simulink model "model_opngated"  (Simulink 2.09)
settings: Solver=ode1  StartTime=0.0  StopTime=1  FixedStep=0.001  MaxStep=0.001  RelTol=1e-5  AbsTol=1e-6
undefined symbols (not defined in the file or in its folder): movedetect

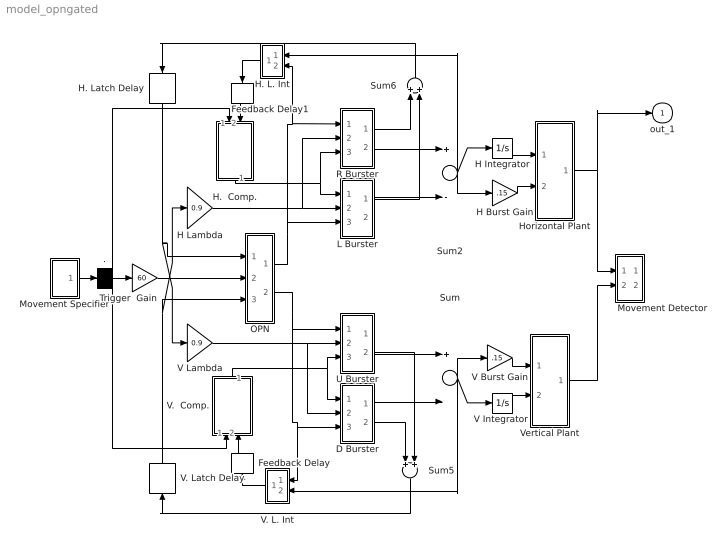
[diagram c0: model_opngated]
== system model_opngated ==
  . : Demux  Outputs=3
  D Burster : Subsystem
  Feedback Delay : TransportDelay  Orientation=up  DelayTime=.005  InitialInput=00  BufferSize=1024
  Feedback Delay1 : TransportDelay  Orientation=down  DelayTime=.005  InitialInput=00  BufferSize=1024
  H Burst Gain : Gain  Gain=.15
  H Integrator : Integrator  ExternalReset=none  InitialConditionSource=internal  InitialCondition=0  LimitOutput=off  UpperSaturationLimit=inf  LowerSaturationLimit=-inf  ShowSaturationPort=off  ShowStatePort=off  AbsoluteTolerance=auto
  H Lambda : Gain  Gain=0.9
  H.  Comp. : Subsystem  Orientation=down
  H. L. Int : Subsystem  Orientation=left
  H. Latch Delay : TransportDelay  Orientation=down  DelayTime=0  InitialInput=00  BufferSize=1024
  Horizontal Plant : Subsystem
  L Burster : Subsystem
  Movement Detector : Subsystem
  Movement Specifier : Subsystem
  OPN : Subsystem
  R Burster : Subsystem
  Sum : Sum  Inputs=+-
  Sum2 : Sum  Inputs=+-
  Sum5 : Sum  Orientation=down  Inputs=++
  Sum6 : Sum  Orientation=up  Inputs=++
  Trigger  Gain : Gain  Gain=60
  U Burster : Subsystem
  V Burst Gain : Gain  Gain=.15
  "V Integrator " : Integrator  ExternalReset=none  InitialConditionSource=internal  InitialCondition=0  LimitOutput=off  UpperSaturationLimit=inf  LowerSaturationLimit=-inf  ShowSaturationPort=off  ShowStatePort=off  AbsoluteTolerance=auto
  V Lambda : Gain  Gain=0.9
  V.  Comp. : Subsystem  Orientation=up
  V. L. Int : Subsystem  Orientation=left
  V. Latch Delay : TransportDelay  Orientation=up  DelayTime=0  InitialInput=00  BufferSize=1024
  Vertical Plant : Subsystem
  out_1 : Outport  Port=1  InitialOutput=0
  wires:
  OPN/1(out_1) -> H. L. Int/2(OPN Input), R Burster/1(in_3), L Burster/3(in_3)
  Horizontal Plant/1(out_1) -> out_1/1, Movement Detector/1(Horizontal Position)
  ./3 -> V.  Comp./1(in_4)
  Movement Specifier/1(out_1) -> ./1
  ./1 -> H.  Comp./1(in_1)
  ./2 -> Trigger  Gain/1
  Vertical Plant/1(out_1) -> Movement Detector/2(Veritcal Position)
  H Integrator/1 -> Horizontal Plant/1(in_1)
  OPN/2(out_4) -> V. L. Int/1(OPN Input), D Burster/3(in_3), U Burster/1(in_3)
  H. Latch Delay/1 -> V Lambda/1, OPN/1(in_1)
  V. Latch Delay/1 -> H Lambda/1, OPN/3(in_3)
  Trigger  Gain/1 -> OPN/2(in_2)
  R Burster/1(out_2) -> Sum6/1
  Sum5/1 -> V. Latch Delay/1
  Sum6/1 -> H. Latch Delay/1
  L Burster/1(out_1) -> Sum6/2
  V.  Comp./1(out_1) -> D Burster/1(in_1), U Burster/3(in_1)
  V Lambda/1 -> D Burster/2(in_2), U Burster/2(in_2)
  D Burster/1(out_2) -> Sum/2
  D Burster/2(out_3) -> Sum5/1
  U Burster/1(out_3) -> Sum/1
  U Burster/2(out_4) -> Sum5/2
  H Lambda/1 -> R Burster/2(in_2), L Burster/2(in_2)
  R Burster/2(out_3) -> Sum2/1
  L Burster/2(out_2) -> Sum2/2
  H.  Comp./1(out_1) -> R Burster/3(in_1), L Burster/1(in_1)
  Sum/1 -> V. L. Int/2(BURST Input), "V Integrator "/1, V Burst Gain/1
  "V Integrator "/1 -> Vertical Plant/2(in_2)
  V Burst Gain/1 -> Vertical Plant/1(in_1)
  Sum2/1 -> H. L. Int/1(BURST Input), H Burst Gain/1, H Integrator/1
  H Burst Gain/1 -> Horizontal Plant/2(in_2)
  V. L. Int/1(out_1) -> Feedback Delay/1
  Feedback Delay/1 -> V.  Comp./2(in_5)
  H. L. Int/1(out_1) -> Feedback Delay1/1
  Feedback Delay1/1 -> H.  Comp./2(in_2)

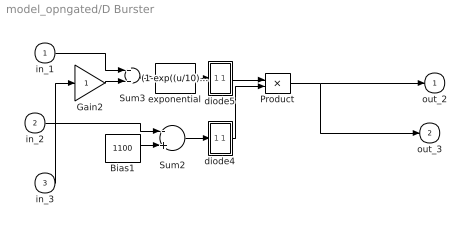
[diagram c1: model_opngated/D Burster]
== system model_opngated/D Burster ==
  in_1 : Inport  Port=1  PortWidth=-1  SampleTime=-1
  in_2 : Inport  Port=2  PortWidth=-1  SampleTime=-1
  in_3 : Inport  Port=3  PortWidth=-1  SampleTime=-1
  Bias1 : Constant  Value=1100
  Gain2 : Gain  Gain=1
  Product : Product  Inputs=2
  Sum2 : Sum  Inputs=-+
  Sum3 : Sum  Inputs=++
  diode4 : Subsystem
  diode5 : Subsystem
  exponential : Fcn  Expr=(1-exp((u/10)))
  out_2 : Outport  Port=1  InitialOutput=0
  out_3 : Outport  Port=2  InitialOutput=0
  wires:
  Product/1 -> out_3/1, out_2/1
  in_3/1 -> Gain2/1
  diode5/1(out_1) -> Product/1
  exponential/1 -> diode5/1(in_1)
  diode4/1(out_1) -> Product/2
  Sum2/1 -> diode4/1(in_1)
  in_2/1 -> Sum2/1
  Bias1/1 -> Sum2/2
  Sum3/1 -> exponential/1
  in_1/1 -> Sum3/1
  Gain2/1 -> Sum3/2

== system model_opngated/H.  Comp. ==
  in_1 : Inport  Port=1  PortWidth=-1  SampleTime=-1
  in_2 : Inport  Port=2  PortWidth=-1  SampleTime=-1
  Sum : Sum  Inputs=+-
  out_1 : Outport  Port=1  InitialOutput=0
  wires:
  in_2/1 -> Sum/2
  in_1/1 -> Sum/1
  Sum/1 -> out_1/1

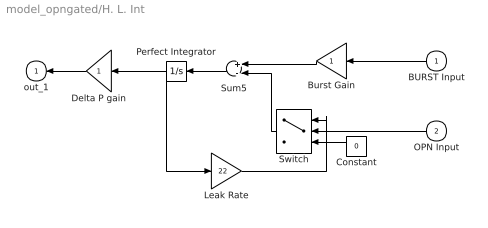
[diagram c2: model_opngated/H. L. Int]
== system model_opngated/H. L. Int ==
  BURST Input : Inport  Orientation=left  Port=1  PortWidth=-1  SampleTime=-1
  OPN Input : Inport  Orientation=left  Port=2  PortWidth=-1  SampleTime=-1
  Burst Gain : Gain  Orientation=left  Gain=1
  Constant : Constant  Orientation=left  Value=0
  Delta P gain : Gain  Orientation=left  Gain=1
  Leak Rate : Gain  Gain=22
  Perfect Integrator : Integrator  Orientation=left  ExternalReset=none  InitialConditionSource=internal  InitialCondition=0  LimitOutput=off  UpperSaturationLimit=inf  LowerSaturationLimit=-inf  ShowSaturationPort=off  ShowStatePort=off  AbsoluteTolerance=auto
  Sum5 : Sum  Orientation=left  Inputs=+-
  Switch : Switch  Orientation=left  Threshold=50
  out_1 : Outport  Orientation=left  Port=1  InitialOutput=0
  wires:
  Switch/1 -> Sum5/2
  Constant/1 -> Switch/3
  Leak Rate/1 -> Switch/1
  Perfect Integrator/1 -> Leak Rate/1, Delta P gain/1
  OPN Input/1 -> Switch/2
  BURST Input/1 -> Burst Gain/1
  Burst Gain/1 -> Sum5/1
  Delta P gain/1 -> out_1/1
  Sum5/1 -> Perfect Integrator/1

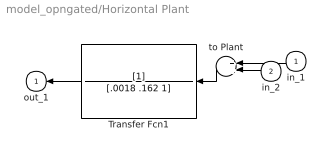
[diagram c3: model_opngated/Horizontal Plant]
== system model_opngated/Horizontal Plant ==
  in_1 : Inport  Orientation=left  Port=1  PortWidth=-1  SampleTime=-1
  in_2 : Inport  Orientation=left  Port=2  PortWidth=-1  SampleTime=-1
  Transfer Fcn1 : TransferFcn  Orientation=left  Numerator=[1]  Denominator=[.0018 .162 1]
  to Plant : Sum  Orientation=left  Inputs=++
  out_1 : Outport  Orientation=left  Port=1  InitialOutput=0
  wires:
  Transfer Fcn1/1 -> out_1/1
  in_2/1 -> to Plant/2
  in_1/1 -> to Plant/1
  to Plant/1 -> Transfer Fcn1/1

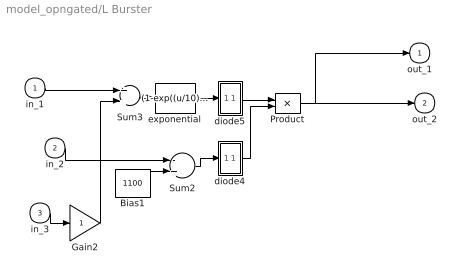
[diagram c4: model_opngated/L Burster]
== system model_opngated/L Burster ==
  in_1 : Inport  Port=1  PortWidth=-1  SampleTime=-1
  in_2 : Inport  Port=2  PortWidth=-1  SampleTime=-1
  in_3 : Inport  Port=3  PortWidth=-1  SampleTime=-1
  Bias1 : Constant  Value=1100
  Gain2 : Gain  Gain=1
  Product : Product  Inputs=2
  Sum2 : Sum  Inputs=-+
  Sum3 : Sum  Inputs=++
  diode4 : Subsystem
  diode5 : Subsystem
  exponential : Fcn  Expr=(1-exp((u/10)))
  out_1 : Outport  Port=1  InitialOutput=0
  out_2 : Outport  Port=2  InitialOutput=0
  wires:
  Product/1 -> out_1/1, out_2/1
  Bias1/1 -> Sum2/2
  in_2/1 -> Sum2/1
  Sum2/1 -> diode4/1(in_1)
  diode4/1(out_1) -> Product/2
  exponential/1 -> diode5/1(in_1)
  diode5/1(out_1) -> Product/1
  Sum3/1 -> exponential/1
  in_3/1 -> Gain2/1
  Gain2/1 -> Sum3/2
  in_1/1 -> Sum3/1

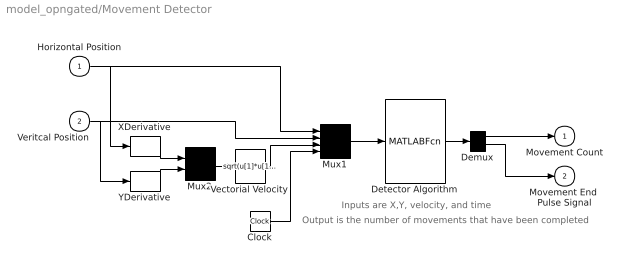
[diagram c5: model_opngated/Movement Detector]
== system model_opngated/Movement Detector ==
  note: Inputs are X,Y, velocity, and time
  note: Output is the number of movements that have been completed
  Horizontal Position : Inport  Port=1  PortWidth=-1  SampleTime=-1
  Veritcal Position : Inport  Port=2  PortWidth=-1  SampleTime=-1
  Clock : Clock
  Demux : Demux  Outputs=2
  Detector Algorithm : MATLABFcn  MATLABFcn=movedetect(u(1),u(2),u(3),u(4))  OutputWidth=2
  Mux1 : Mux  Inputs=4
  Mux2 : Mux  Inputs=2
  Vectorial Velocity : Fcn  Expr=sqrt(u[1]*u[1]+u[2]*u[2])
  XDerivative : Derivative
  YDerivative : Derivative
  Movement Count : Outport  Port=1  InitialOutput=0
  Movement End  Pulse Signal : Outport  Port=2  InitialOutput=0
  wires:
  Demux/2 -> Movement End  Pulse Signal/1
  Demux/1 -> Movement Count/1
  Detector Algorithm/1 -> Demux/1
  Horizontal Position/1 -> XDerivative/1, Mux1/1
  Veritcal Position/1 -> YDerivative/1, Mux1/2
  Vectorial Velocity/1 -> Mux1/3
  Clock/1 -> Mux1/4
  Mux2/1 -> Vectorial Velocity/1
  XDerivative/1 -> Mux2/1
  YDerivative/1 -> Mux2/2
  Mux1/1 -> Detector Algorithm/1

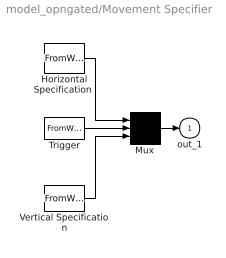
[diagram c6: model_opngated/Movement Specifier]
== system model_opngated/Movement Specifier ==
  "Horizontal Specification " : FromWorkspace  VariableName=hspec
  Mux : Mux  Inputs=3
  Trigger : FromWorkspace  VariableName=trigspec
  Vertical Specification : FromWorkspace  VariableName=vspec
  out_1 : Outport  Port=1  InitialOutput=0
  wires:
  Mux/1 -> out_1/1
  Trigger/1 -> Mux/2
  "Horizontal Specification "/1 -> Mux/1
  Vertical Specification/1 -> Mux/3

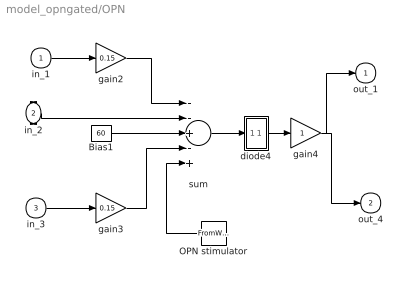
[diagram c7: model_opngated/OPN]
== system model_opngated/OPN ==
  in_1 : Inport  Port=1  PortWidth=-1  SampleTime=-1
  in_2 : Inport  Port=2  PortWidth=-1  SampleTime=-1
  in_3 : Inport  Port=3  PortWidth=-1  SampleTime=-1
  Bias1 : Constant  Value=60
  OPN stimulator : FromWorkspace  Orientation=left  VariableName=stimulate
  diode4 : Subsystem
  gain2 : Gain  Gain=0.15
  gain3 : Gain  Gain=0.15
  gain4 : Gain  Gain=1
  sum : Sum  Inputs=--+-+
  out_1 : Outport  Port=1  InitialOutput=0
  out_4 : Outport  Port=2  InitialOutput=0
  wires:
  OPN stimulator/1 -> sum/5
  gain4/1 -> out_4/1, out_1/1
  diode4/1(out_1) -> gain4/1
  gain3/1 -> sum/4
  in_3/1 -> gain3/1
  gain2/1 -> sum/1
  in_1/1 -> gain2/1
  Bias1/1 -> sum/3
  in_2/1 -> sum/2
  sum/1 -> diode4/1(in_1)

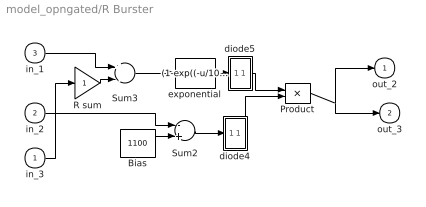
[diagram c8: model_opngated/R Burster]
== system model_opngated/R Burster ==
  in_3 : Inport  Port=1  PortWidth=-1  SampleTime=-1
  in_2 : Inport  Port=2  PortWidth=-1  SampleTime=-1
  in_1 : Inport  Port=3  PortWidth=-1  SampleTime=-1
  Bias : Constant  Value=1100
  Product : Product  Inputs=2
  R sum : Gain  Gain=1
  Sum2 : Sum  Inputs=-+
  Sum3 : Sum  Inputs=+-
  diode4 : Subsystem
  diode5 : Subsystem
  exponential : Fcn  Expr=(1-exp((-u/10)))
  out_2 : Outport  Port=1  InitialOutput=0
  out_3 : Outport  Port=2  InitialOutput=0
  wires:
  in_3/1 -> R sum/1
  Product/1 -> out_3/1, out_2/1
  Bias/1 -> Sum2/2
  in_2/1 -> Sum2/1
  Sum2/1 -> diode4/1(in_1)
  diode4/1(out_1) -> Product/2
  exponential/1 -> diode5/1(in_1)
  diode5/1(out_1) -> Product/1
  R sum/1 -> Sum3/2
  in_1/1 -> Sum3/1
  Sum3/1 -> exponential/1

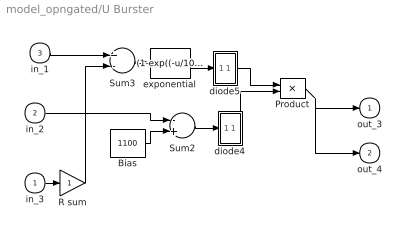
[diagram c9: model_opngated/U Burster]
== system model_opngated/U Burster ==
  in_3 : Inport  Port=1  PortWidth=-1  SampleTime=-1
  in_2 : Inport  Port=2  PortWidth=-1  SampleTime=-1
  in_1 : Inport  Port=3  PortWidth=-1  SampleTime=-1
  Bias : Constant  Value=1100
  Product : Product  Inputs=2
  R sum : Gain  Gain=1
  Sum2 : Sum  Inputs=-+
  Sum3 : Sum  Inputs=+-
  diode4 : Subsystem
  diode5 : Subsystem
  exponential : Fcn  Expr=(1-exp((-u/10)))
  out_3 : Outport  Port=1  InitialOutput=0
  out_4 : Outport  Port=2  InitialOutput=0
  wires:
  Product/1 -> out_3/1, out_4/1
  in_3/1 -> R sum/1
  Bias/1 -> Sum2/2
  in_2/1 -> Sum2/1
  Sum2/1 -> diode4/1(in_1)
  diode4/1(out_1) -> Product/2
  exponential/1 -> diode5/1(in_1)
  diode5/1(out_1) -> Product/1
  in_1/1 -> Sum3/1
  R sum/1 -> Sum3/2
  Sum3/1 -> exponential/1

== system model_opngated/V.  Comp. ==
  in_4 : Inport  Port=1  PortWidth=-1  SampleTime=-1
  in_5 : Inport  Port=2  PortWidth=-1  SampleTime=-1
  Sum : Sum  Inputs=-+
  out_1 : Outport  Port=1  InitialOutput=0
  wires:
  in_4/1 -> Sum/2
  in_5/1 -> Sum/1
  Sum/1 -> out_1/1

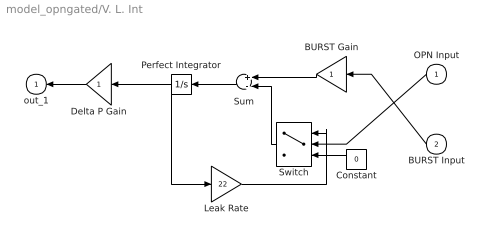
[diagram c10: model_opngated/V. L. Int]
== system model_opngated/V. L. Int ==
  OPN Input : Inport  Orientation=left  Port=1  PortWidth=-1  SampleTime=-1
  BURST Input : Inport  Orientation=left  Port=2  PortWidth=-1  SampleTime=-1
  BURST Gain : Gain  Orientation=left  Gain=1
  Constant : Constant  Orientation=left  Value=0
  Delta P Gain : Gain  Orientation=left  Gain=1
  Leak Rate : Gain  Gain=22
  Perfect Integrator : Integrator  Orientation=left  ExternalReset=none  InitialConditionSource=internal  InitialCondition=0  LimitOutput=off  UpperSaturationLimit=inf  LowerSaturationLimit=-inf  ShowSaturationPort=off  ShowStatePort=off  AbsoluteTolerance=auto
  Sum : Sum  Orientation=left  Inputs=+-
  Switch : Switch  Orientation=left  Threshold=50
  out_1 : Outport  Orientation=left  Port=1  InitialOutput=0
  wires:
  BURST Input/1 -> BURST Gain/1
  OPN Input/1 -> Switch/2
  Sum/1 -> Perfect Integrator/1
  Perfect Integrator/1 -> Delta P Gain/1, Leak Rate/1
  Delta P Gain/1 -> out_1/1
  BURST Gain/1 -> Sum/1
  Leak Rate/1 -> Switch/1
  Constant/1 -> Switch/3
  Switch/1 -> Sum/2

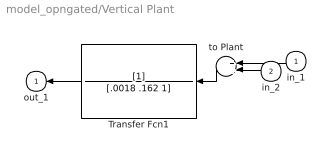
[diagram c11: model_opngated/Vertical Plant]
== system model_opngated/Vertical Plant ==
  in_1 : Inport  Orientation=left  Port=1  PortWidth=-1  SampleTime=-1
  in_2 : Inport  Orientation=left  Port=2  PortWidth=-1  SampleTime=-1
  Transfer Fcn1 : TransferFcn  Orientation=left  Numerator=[1]  Denominator=[.0018 .162 1]
  to Plant : Sum  Orientation=left  Inputs=++
  out_1 : Outport  Orientation=left  Port=1  InitialOutput=0
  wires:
  Transfer Fcn1/1 -> out_1/1
  in_2/1 -> to Plant/2
  in_1/1 -> to Plant/1
  to Plant/1 -> Transfer Fcn1/1

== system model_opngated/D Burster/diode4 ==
  in_1 : Inport  Port=1  PortWidth=-1  SampleTime=-1
  Switch : Switch  Threshold=0
  diode1 : Constant  Value=0
  out_1 : Outport  Port=1  InitialOutput=0
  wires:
  diode1/1 -> Switch/3
  Switch/1 -> out_1/1
  in_1/1 -> Switch/1, Switch/2

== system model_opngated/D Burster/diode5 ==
  in_1 : Inport  Port=1  PortWidth=-1  SampleTime=-1
  Switch : Switch  Threshold=0
  diode1 : Constant  Value=0
  out_1 : Outport  Port=1  InitialOutput=0
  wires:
  diode1/1 -> Switch/3
  Switch/1 -> out_1/1
  in_1/1 -> Switch/1, Switch/2

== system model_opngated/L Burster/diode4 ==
  in_1 : Inport  Port=1  PortWidth=-1  SampleTime=-1
  Switch : Switch  Threshold=0
  diode1 : Constant  Value=0
  out_1 : Outport  Port=1  InitialOutput=0
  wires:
  in_1/1 -> Switch/1, Switch/2
  Switch/1 -> out_1/1
  diode1/1 -> Switch/3

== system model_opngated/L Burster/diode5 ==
  in_1 : Inport  Port=1  PortWidth=-1  SampleTime=-1
  Switch : Switch  Threshold=0
  diode1 : Constant  Value=0
  out_1 : Outport  Port=1  InitialOutput=0
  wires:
  in_1/1 -> Switch/1, Switch/2
  Switch/1 -> out_1/1
  diode1/1 -> Switch/3

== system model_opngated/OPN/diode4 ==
  in_1 : Inport  Port=1  PortWidth=-1  SampleTime=-1
  Switch : Switch  Threshold=0
  diode1 : Constant  Value=0
  out_1 : Outport  Port=1  InitialOutput=0
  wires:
  in_1/1 -> Switch/2, Switch/1
  Switch/1 -> out_1/1
  diode1/1 -> Switch/3

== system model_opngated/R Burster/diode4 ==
  in_1 : Inport  Port=1  PortWidth=-1  SampleTime=-1
  Switch : Switch  Threshold=0
  diode1 : Constant  Value=0
  out_1 : Outport  Port=1  InitialOutput=0
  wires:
  diode1/1 -> Switch/3
  Switch/1 -> out_1/1
  in_1/1 -> Switch/1, Switch/2

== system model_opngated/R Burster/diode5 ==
  in_1 : Inport  Port=1  PortWidth=-1  SampleTime=-1
  Switch : Switch  Threshold=0
  diode1 : Constant  Value=0
  out_1 : Outport  Port=1  InitialOutput=0
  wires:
  in_1/1 -> Switch/1, Switch/2
  Switch/1 -> out_1/1
  diode1/1 -> Switch/3

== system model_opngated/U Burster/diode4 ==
  in_1 : Inport  Port=1  PortWidth=-1  SampleTime=-1
  Switch : Switch  Threshold=0
  diode1 : Constant  Value=0
  out_1 : Outport  Port=1  InitialOutput=0
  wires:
  diode1/1 -> Switch/3
  Switch/1 -> out_1/1
  in_1/1 -> Switch/1, Switch/2

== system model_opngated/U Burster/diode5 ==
  in_1 : Inport  Port=1  PortWidth=-1  SampleTime=-1
  Switch : Switch  Threshold=0
  diode1 : Constant  Value=0
  out_1 : Outport  Port=1  InitialOutput=0
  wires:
  in_1/1 -> Switch/1, Switch/2
  Switch/1 -> out_1/1
  diode1/1 -> Switch/3
